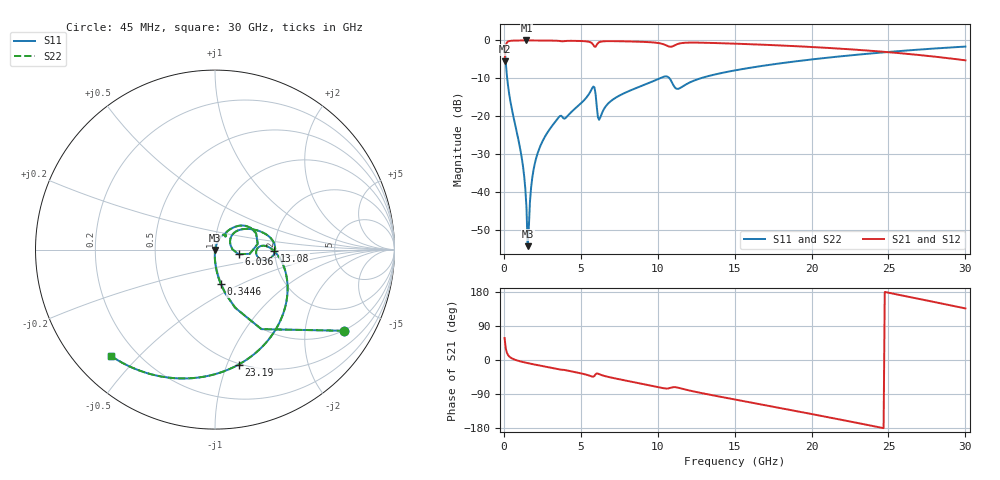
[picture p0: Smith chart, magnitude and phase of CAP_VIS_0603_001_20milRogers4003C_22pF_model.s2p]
! S-parameter model data by Modelithics Inc.  support@modelithics.com  813-866-6335  Tampa FL USA
! S-Parameter data specifications:
! Substrate: 20-mil Rogers 4003C, substrate thickness, H=0.508mm, Dielectric constant, Er=3.75
! PCB Mounting Pad Footprint: Pad width, PadW=0.90mm , Pad length, PadL=1.00mm , Pad gap, PadG (edge-to-edge)=1.00mm , Reference planes=3.0mm apart
! Created Wed Nov 18 13:27:23 2015
# hz S ma R 50
! 2 Port Network Data from SP1.SP block
! freq  magS11  angS11  magS21  angS21  magS12  angS12  magS22  angS22
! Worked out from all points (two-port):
!   401 points, 45 MHz to 30 GHz, reference 50 ohm
!   highest |S21| = -0.01 dB at 1.468 GHz (marker M1); lowest = -5.5 dB at 45 MHz (marker M2)
!   |S21| within 3 dB of the highest: 89.79 MHz to 24.72 GHz (24.63 GHz wide, 199 % of centre)
!   lowest |S11| = -54.3 dB at 1.543 GHz (marker M3), VSWR 1.00, Z = 50.1 - j0.156 ohm
!   |S11| at or under -10 dB: 213.9 MHz to 10.13 GHz (9.912 GHz wide, 192 % of centre); 10.76 GHz to 12.78 GHz (2.02 GHz wide, 17.2 % of centre)
!   |S22| runs from -54.3 to -1.4 dB; largest |S21 - S12| = 0
!   S11 on the Smith chart (normalised r, x): 45 MHz: 0.99, -3.18; 344.6 MHz: 0.99, -0.40; 6.036 GHz: 1.30, -0.07; 13.08 GHz: 1.98, -0.03; 23.19 GHz: 0.49, -1.10; 30 GHz: 0.11, -0.42
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4.5e7  0.848 -32.2  0.5298 57.8  0.5298 57.8  0.848 -32.2
3.4455e8  0.1952 -80.4  0.9801 9.4  0.9801 9.4  0.1952 -80.4
1.168312e9  0.02753 -92.2  0.9984 -4.7  0.9984 -4.7  0.02753 -92.2
1.467862e9  0.006157 -85.2  0.9985 -7.5  0.9985 -7.5  0.006157 -85.2
1.54275e9  0.00193 -54.0  0.9985 -8.2  0.9985 -8.2  0.00193 -54.0
1.692525e9  0.007411 69.5  0.9984 -9.5  0.9984 -9.5  0.007411 69.5
1.992075e9  0.02291 74.2  0.998 -12.0  0.998 -12.0  0.02291 74.2
2.516288e9  0.0471 71.6  0.9968 -16.2  0.9968 -16.2  0.0471 71.6
3.564712e9  0.09694 59.9  0.9858 -24.6  0.9858 -24.6  0.09694 59.9
5.062462e9  0.1517 51.6  0.9811 -35.8  0.9811 -35.8  0.1517 51.6
5.73645e9  0.2339 31.0  0.9119 -43.7  0.9119 -43.7  0.2339 31.0
6.036e9  0.134 -11.0  0.8759 -35.4  0.8759 -35.4  0.134 -11.0
6.260662e9  0.09574 29.0  0.9589 -38.5  0.9589 -38.5  0.09574 29.0
7.2342e9  0.1739 39.0  0.9768 -48.6  0.9768 -48.6  0.1739 39.0
1.007992e10  0.3133 12.7  0.9203 -72.0  0.9203 -72.0  0.3133 12.7
1.135301e10  0.2305 -1.1  0.9042 -73.3  0.9042 -73.3  0.2305 -1.1
1.307542e10  0.3293 -1.3  0.9306 -89.2  0.9306 -89.2  0.3293 -1.3
1.50225e10  0.4025 -15.5  0.9059 -104.3  0.9059 -104.3  0.4025 -15.5
2.003996e10  0.5619 -53.5  0.818 -142.9  0.818 -142.9  0.5619 -53.5
2.318524e10  0.6538 -78.3  0.7466 -167.7  0.7466 -167.7  0.6538 -78.3
2.505742e10  0.7058 -93.5  0.6976 177.1  0.6976 177.1  0.7058 -93.5
3e10  0.8288 -134.4  0.5459 136.1  0.5459 136.1  0.8288 -134.4
